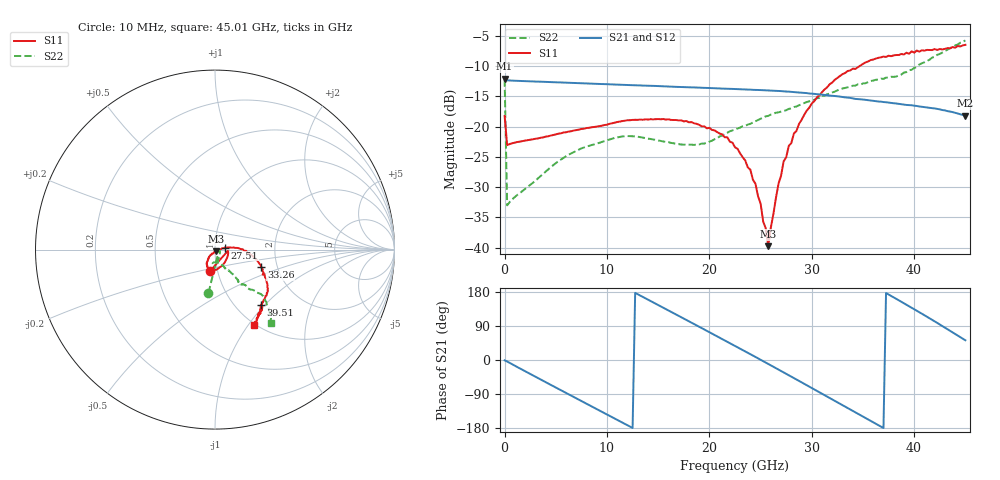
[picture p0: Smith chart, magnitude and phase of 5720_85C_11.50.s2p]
! Device:  ADRF5720
! Description: 0.5dB LSB GaAs MMIC 6-bit Digital Attenuator
! Frequency:  0.000009 -  40 GHz
! Ports:
!	RF1	= Port 1
!	RF2	= Port 2
! Vdd:  3.3 Volt
! Vss:  -3.3 Volt
! Control:  0/3.3 Volt
! State:  11.50 dB attenuation
! Data:  The device was measured using G-S-G Probes on a matrix board.
!  Data was collected using an calibrated 4 port network analyzer.
!  The reference plane for this measurement is at the launchers.
! Note:  Analog Devices supplies this data as a sample of measured data
!  for this product.  Your particular data for this product may vary.
!  Data was taken at 85 degrees C.
!  Analog Devices reserves the right to change this data at anytime.
# GHZ S DB R 45.0
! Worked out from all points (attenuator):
!   181 points, 10 MHz to 45.01 GHz, reference 45 ohm
!   highest |S21| = -12.07 dB at 10 MHz (marker M1); lowest = -18.2 dB at 45.01 GHz (marker M2)
!   lowest |S11| = -39.8 dB at 25.76 GHz (marker M3), VSWR 1.02, Z = 45.4 - j0.823 ohm
!   |S11| at or under -10 dB: start of sweep to 34.69 GHz
!   |S22| runs from -33.0 to -5.8 dB; largest |S21 - S12| = 0.0012
!   S11 on the Smith chart (normalised r, x): 10 MHz: 0.92, -0.22; 27.51 GHz: 1.12, +0.03; 33.26 GHz: 1.65, -0.35; 39.51 GHz: 1.30, -0.95; 45.01 GHz: 0.98, -1.06
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0.01  -18.24 -102.8  -12.07 -0.9  -12.06 -0.9  -12.23 -98.6
0.26  -23.08 -8.3  -12.36 -4.0  -12.36 -4.0  -33.02 -20.9
4.26  -21.61 -39.4  -12.63 -61.9  -12.62 -61.9  -27.10 -57.4
7.76  -20.36 -63.9  -12.86 -111.8  -12.84 -111.8  -23.46 -78.8
11.51  -19.09 -84.7  -13.10 -165.1  -13.09 -165.0  -21.63 -94.3
15.26  -18.80 -101.7  -13.32 141.4  -13.31 141.6  -22.37 -99.1
19.01  -19.72 -114.9  -13.56 87.8  -13.55 87.9  -22.96 -81.6
21.76  -21.78 -122.8  -13.75 48.1  -13.74 48.3  -21.03 -68.0
22.76  -23.68 -124.4  -13.82 33.6  -13.80 33.8  -20.32 -64.9
24.51  -29.45 -123.9  -13.94 8.1  -13.93 8.3  -19.12 -62.6
25.51  -36.82 -82.3  -14.01 -6.7  -13.99 -6.4  -18.31 -61.6
25.76  -39.77 -61.9  -14.03 -10.4  -14.01 -10.2  -18.24 -60.5
26.76  -29.44 4.3  -14.12 -25.3  -14.11 -25.0  -17.65 -58.4
27.26  -25.74 8.3  -14.18 -32.8  -14.16 -32.5  -17.40 -57.7
27.51  -25.08 11.8  -14.21 -36.5  -14.19 -36.2  -17.30 -56.6
28.26  -21.16 8.1  -14.31 -47.8  -14.29 -47.5  -16.78 -56.5
30.26  -15.79 -2.4  -14.60 -77.8  -14.58 -77.6  -15.60 -54.2
33.26  -11.16 -21.0  -15.18 -123.1  -15.16 -122.8  -13.62 -53.0
37.76  -8.37 -42.6  -16.11 168.9  -16.08 169.3  -11.77 -50.1
39.51  -7.98 -50.2  -16.46 142.0  -16.44 142.4  -10.68 -49.0
42.26  -7.33 -55.6  -17.08 97.9  -17.05 98.2  -8.14 -44.6
45.01  -6.49 -63.1  -18.20 52.0  -18.18 52.4  -5.77 -52.9
